| TEXAS INSTRUMENTS INCORPORATED
| Standard Linear and Logic Group
| IBIS Model of SN74ALVCH162244
| 16-BIT BUFFER/DRIVER WITH 3-STATE OUTPUTS
| This file contains package information for the following:
|  SSOP 48-pin (DL) package as [Component] ALVCH162244_DL
|  TSSOP 48-pin (DGG) package as [Component] ALVCH162244_DGG
| This device can be powered at the following Vccs:
|  3.3 volt Vcc
|  2.5 volt Vcc
|  1.8 volt Vcc
| This file provides unique models under the [Model Selector] for each Vcc.
| For operation at a specific Vcc, select the appropriate model after each
| [Model Selector] keyword.
[IBIS Ver]   3.2
[Comment char]  |_char
[File Name]   sn74alvch162244.ibs
[File Rev]   1.1 | b_die
[Date]   February 20, 2002
[Source]   Data created from TI-SPICE simulations at TI-SLL.
[Notes]   The following is an IBIS list for the ALVCH162244.
   Please contact sllibis@ti.com with questions and
   comments concerning SLL IBIS models.
   This IBIS model is created from a BA (back annotated netlist
   Non Monotonic data in input due bus hold
[Disclaimer] Property of Texas Instruments Incorporated.  Unauthorized
   reproduction and/or distribution is strictly prohibited.
   This product is protected under copyright law.
   Created  2002, (C) Copyright  2002, Texas Instruments
   Incorporated, All Rights Reserved
   UNLESS THERE IS A SIGNED, WRITTEN AGREEMENT TO THE
   CONTRARY, TEXAS INSTRUMENTS (TI) IS PROVIDING THE IBIS
   MODELS  AND WITHOUT ANY WARRANTY, EXPRESSED OR
   IMPLIED.  TI assumes no liability for:
   1) the accuracy of the IBIS models provided to your
   company;
   2) the proper functioning of these IBIS Models in your
   design or for any resulting applications; or
   3) infringement of patents, copyrights or intellectual
   property rights resulting from your use of these IBIS
   models.
   TI provides IBIS Models as a service to our customers.
   You and your company shall not distribute, sell or give
   these models to anyone else without prior written
   permission from TI.
   TI reserves the right to make changes to our products or
   to discontinue any semiconductor product or service
   without notice, and advises our customers to obtain the
   latest version of relevant information to verify, before
   placing orders, that the information being relied on is
   current.
   Please be aware that your receipt and use of the IBIS
   information provided shall serve as acceptance of these
   terms and conditions.  If you do not accept these terms,
   you should return or destroy the IBIS models and any
   other accompanying information immediately.
| Component ALVCH162244_DL 48-pin SSOP
[Component]   ALVCH162244_DL
[Manufacturer]   Texas Instruments, Inc.
[Package]
|   typ   min   max
R_pkg   4.800e-02   3.800e-02   5.300e-02
L_pkg   6.046e-09   5.084e-09   7.968e-09
C_pkg   8.130e-13   5.690e-13   1.157e-12
[Pin]   signal_name   model_name   R_pin   L_pin   C_pin
1   1OE_BAR   ALVCH162244_NOE   4.600e-02   7.968e-09   1.017e-12
2   1Y1   ALVCH162244_OUT   4.400e-02   7.299e-09   1.157e-12
3   1Y2   ALVCH162244_OUT   4.300e-02   6.765e-09   1.058e-12
4   GND   GND   4.100e-02   6.269e-09   9.330e-13
5   1Y3   ALVCH162244_OUT   3.800e-02   5.856e-09   8.290e-13
6   1Y4   ALVCH162244_OUT   4.600e-02   5.802e-09   7.900e-13
7   VCC   POWER   5.000e-02   5.656e-09   7.380e-13
8   2Y1   ALVCH162244_OUT   5.300e-02   5.500e-09   6.430e-13
9   2Y2   ALVCH162244_OUT   5.200e-02   5.304e-09   6.060e-13
10   GND   GND   5.300e-02   5.189e-09   5.830e-13
11   2Y3   ALVCH162244_OUT   5.100e-02   5.084e-09   5.690e-13
12   2Y4   ALVCH162244_OUT   5.300e-02   5.862e-09   8.330e-13
13   3Y1   ALVCH162244_OUT   5.300e-02   5.862e-09   8.330e-13
14   3Y2   ALVCH162244_OUT   5.100e-02   5.084e-09   5.690e-13
15   GND   GND   5.300e-02   5.189e-09   5.830e-13
16   3Y3   ALVCH162244_OUT   5.200e-02   5.304e-09   6.060e-13
17   3Y4   ALVCH162244_OUT   5.300e-02   5.500e-09   6.430e-13
18   VCC   POWER   5.000e-02   5.656e-09   7.380e-13
19   4Y1   ALVCH162244_OUT   4.600e-02   5.802e-09   7.900e-13
20   4Y2   ALVCH162244_OUT   3.800e-02   5.856e-09   8.290e-13
21   GND   GND   4.100e-02   6.269e-09   9.330e-13
22   4Y3   ALVCH162244_OUT   4.300e-02   6.765e-09   1.058e-12
23   4Y4   ALVCH162244_OUT   4.400e-02   7.299e-09   1.157e-12
24   4OE_BAR   ALVCH162244_NOE   4.600e-02   7.968e-09   1.017e-12
25   3OE_BAR   ALVCH162244_NOE   4.600e-02   7.968e-09   1.017e-12
26   4A4   ALVCH162244_IN   4.400e-02   7.299e-09   1.157e-12
27   4A3   ALVCH162244_IN   4.300e-02   6.765e-09   1.058e-12
28   GND   GND   4.100e-02   6.269e-09   9.330e-13
29   4A2   ALVCH162244_IN   3.800e-02   5.856e-09   8.290e-13
30   4A1   ALVCH162244_IN   4.600e-02   5.802e-09   7.900e-13
31   VCC   POWER   5.000e-02   5.656e-09   7.380e-13
32   3A4   ALVCH162244_IN   5.300e-02   5.500e-09   6.430e-13
33   3A3   ALVCH162244_IN   5.200e-02   5.304e-09   6.060e-13
34   GND   GND   5.300e-02   5.189e-09   5.830e-13
35   3A2   ALVCH162244_IN   5.100e-02   5.084e-09   5.690e-13
36   3A1   ALVCH162244_IN   5.300e-02   5.862e-09   8.330e-13
37   2A4   ALVCH162244_IN   5.300e-02   5.862e-09   8.330e-13
38   2A3   ALVCH162244_IN   5.100e-02   5.084e-09   5.690e-13
39   GND   GND   5.300e-02   5.189e-09   5.830e-13
40   2A2   ALVCH162244_IN   5.200e-02   5.304e-09   6.060e-13
41   2A1   ALVCH162244_IN   5.300e-02   5.500e-09   6.430e-13
42   VCC   POWER   5.000e-02   5.656e-09   7.380e-13
43   1A4   ALVCH162244_IN   4.600e-02   5.802e-09   7.900e-13
44   1A3   ALVCH162244_IN   3.800e-02   5.856e-09   8.290e-13
45   GND   GND   4.100e-02   6.269e-09   9.330e-13
46   1A2   ALVCH162244_IN   4.300e-02   6.765e-09   1.058e-12
47   1A1   ALVCH162244_IN   4.400e-02   7.299e-09   1.157e-12
48   2OE_BAR   ALVCH162244_NOE   4.600e-02   7.967e-09   1.017e-12
| Component ALVCH162244_DGG 48-pin TSSOP
[Component]   ALVCH162244_DGG
[Manufacturer]   Texas Instruments, Inc.
[Package]
|   typ   min   max
R_pkg   4.400e-02   3.800e-02   5.100e-02
L_pkg   3.019e-09   2.486e-09   4.099e-09
C_pkg   5.070e-13   3.340e-13   8.090e-13
[Pin]   signal_name   model_name   R_pin   L_pin   C_pin
1   1OE_BAR   ALVCH162244_NOE   4.100e-02   4.017e-09   7.590e-13
2   1Y1   ALVCH162244_OUT   4.200e-02   3.737e-09   7.920e-13
3   1Y2   ALVCH162244_OUT   4.200e-02   3.480e-09   6.610e-13
4   GND   GND   3.800e-02   3.131e-09   5.750e-13
5   1Y3   ALVCH162244_OUT   4.700e-02   3.122e-09   5.660e-13
6   1Y4   ALVCH162244_OUT   4.300e-02   2.948e-09   5.040e-13
7   VCC   POWER   4.500e-02   2.845e-09   3.970e-13
8   2Y1   ALVCH162244_OUT   4.900e-02   2.835e-09   3.940e-13
9   2Y2   ALVCH162244_OUT   4.800e-02   2.715e-09   3.780e-13
10   GND   GND   5.000e-02   2.664e-09   3.630e-13
11   2Y3   ALVCH162244_OUT   5.000e-02   2.585e-09   3.480e-13
12   2Y4   ALVCH162244_OUT   4.900e-02   2.550e-09   3.370e-13
13   3Y1   ALVCH162244_OUT   4.900e-02   2.541e-09   3.360e-13
14   3Y2   ALVCH162244_OUT   5.000e-02   2.574e-09   3.480e-13
15   GND   GND   4.900e-02   2.618e-09   3.590e-13
16   3Y3   ALVCH162244_OUT   4.600e-02   2.671e-09   3.750e-13
17   3Y4   ALVCH162244_OUT   4.500e-02   2.754e-09   3.890e-13
18   VCC   POWER   4.400e-02   2.823e-09   4.500e-13
19   4Y1   ALVCH162244_OUT   4.200e-02   2.968e-09   5.030e-13
20   4Y2   ALVCH162244_OUT   5.100e-02   3.108e-09   5.350e-13
21   GND   GND   4.200e-02   3.175e-09   5.870e-13
22   4Y3   ALVCH162244_OUT   4.100e-02   3.449e-09   6.780e-13
23   4Y4   ALVCH162244_OUT   4.400e-02   3.766e-09   8.040e-13
24   40E_BAR   ALVCH162244_NOE   4.300e-02   4.065e-09   7.610e-13
25   30E_BAR   ALVCH162244_NOE   4.100e-02   3.994e-09   7.570e-13
26   4A4   ALVCH162244_IN   3.900e-02   3.649e-09   7.890e-13
27   4A3   ALVCH162244_IN   3.800e-02   3.362e-09   6.600e-13
28   GND   GND   3.800e-02   3.082e-09   5.740e-13
29   4A2   ALVCH162244_IN   4.400e-02   2.990e-09   5.220e-13
30   4A1   ALVCH162244_IN   4.100e-02   2.917e-09   4.950e-13
31   VCC   POWER   4.300e-02   2.820e-09   4.480e-13
32   3A4   ALVCH162244_IN   4.300e-02   2.699e-09   3.850e-13
33   3A3   ALVCH162244_IN   4.500e-02   2.628e-09   3.720e-13
34   GND   GND   4.600e-02   2.556e-09   3.560e-13
35   3A2   ALVCH162244_IN   4.600e-02   2.495e-09   3.440e-13
36   3A1   ALVCH162244_IN   4.700e-02   2.487e-09   3.340e-13
37   2A4   ALVCH162244_IN   4.700e-02   2.490e-09   3.350e-13
38   2A3   ALVCH162244_IN   4.600e-02   2.486e-09   3.430e-13
39   GND   GND   4.500e-02   2.566e-09   3.560e-13
40   2A2   ALVCH162244_IN   4.400e-02   2.639e-09   3.740e-13
41   2A1   ALVCH162244_IN   4.300e-02   2.701e-09   3.860e-13
42   VCC   POWER   4.300e-02   2.817e-09   4.500e-13
43   1A4   ALVCH162244_IN   4.100e-02   2.935e-09   5.010e-13
44   1A3   ALVCH162244_IN   4.700e-02   3.035e-09   5.290e-13
45   GND   GND   4.300e-02   3.171e-09   5.890e-13
46   1A2   ALVCH162244_IN   4.000e-02   3.415e-09   6.820e-13
47   1A1   ALVCH162244_IN   4.300e-02   3.741e-09   8.090e-13
48   2OE_BAR   ALVCH162244_NOE   4.400e-02   4.099e-09   7.640e-13
| Model ALVCH162244_IN
[Model Selector]   ALVCH162244_IN
ALVCH162244_IN_33   3.3 volt Vcc
ALVCH162244_IN_25   2.5 volt Vcc
ALVCH162244_IN_18   1.8 volt Vcc
| Model ALVCH162244_NOE
[Model Selector]   ALVCH162244_NOE
ALVCH162244_NOE_33   3.3 volt Vcc
ALVCH162244_NOE_25   2.5 volt Vcc
ALVCH162244_NOE_18   1.8 volt Vcc
| Model ALVCH162244_OUT
[Model Selector]   ALVCH162244_OUT
ALVCH162244_OUT_33   3.3 volt Vcc
ALVCH162244_OUT_25   2.5 volt Vcc
ALVCH162244_OUT_18   1.8 volt Vcc
| Models and submodels in the file (9): ALVCH162244_IN_33 (Input), ALVCH162244_IN_25 (Input), ALVCH162244_IN_18 (Input), ALVCH162244_NOE_33 (Input), ALVCH162244_NOE_25 (Input), ALVCH162244_NOE_18 (Input), ALVCH162244_OUT_33 (3-state), ALVCH162244_OUT_25 (3-state), ALVCH162244_OUT_18 (3-state)
